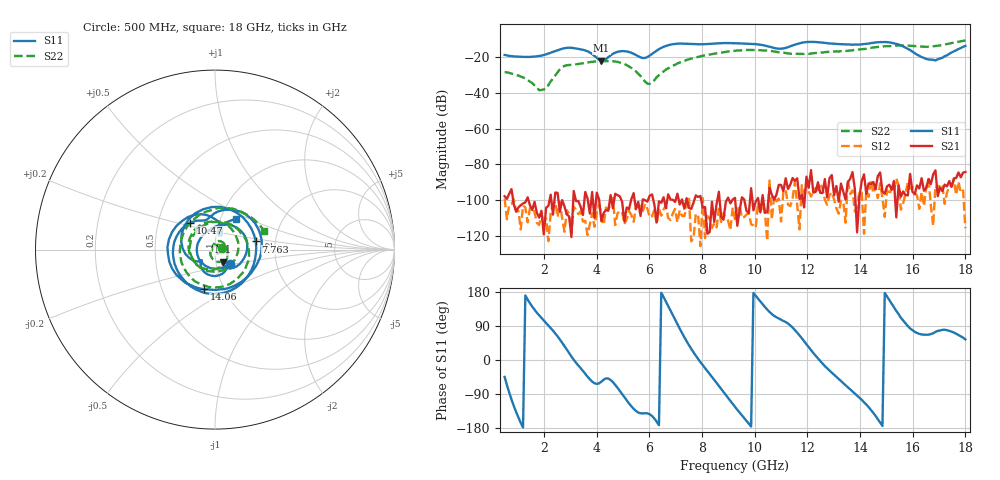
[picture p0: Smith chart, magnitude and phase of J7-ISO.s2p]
!Agilent Technologies,N5230A,MY45001360,A.07.50.67
!Agilent N5230A: A.07.50.67
!Date: Tuesday, April 16, 2024 16:03:02
!Correction: S11(Full 2 Port(1,2))
!S21(Full 2 Port(1,2))
!S12(Full 2 Port(1,2))
!S22(Full 2 Port(1,2))
!S2P File: Measurements: S11, S21, S12, S22:
# Hz S  dB  R 50
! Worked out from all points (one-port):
!   201 points, 500 MHz to 18 GHz, reference 50 ohm
!   lowest |S11| = -22.0 dB at 4.175 GHz (marker M1), VSWR 1.17, Z = 54 - j7.27 ohm
!   |S11| at or under -10 dB: start of sweep to end of sweep
!   S11 on the Smith chart (normalised r, x): 500 MHz: 1.16, -0.19; 7.763 GHz: 1.58, +0.15; 10.47 GHz: 0.73, +0.23; 14.06 GHz: 0.81, -0.38; 18 GHz: 1.19, +0.42
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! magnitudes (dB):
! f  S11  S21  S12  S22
! 500 MHz  -18.7  -97.8  -99.1  -28.4
! 1.288 GHz  -19.9  -101.3  -104.1  -31.9
! 1.9 GHz  -19.1  -106.0  -107.8  -38.4
! 2.075 GHz  -18.4  -104.3  -110.1  -37.7
! 2.688 GHz  -15.3  -100.0  -110.2  -25.6
! 3.475 GHz  -15.9  -108.3  -112.0  -23.4
! 4.175 GHz  -22.0  -111.8  -107.4  -22.3
! 4.7 GHz  -17.5  -96.4  -113.9  -22.4
! 5.05 GHz  -16.7  -111.9  -113.4  -23.8
! 5.487 GHz  -18.8  -105.1  -104.3  -27.9
! 5.925 GHz  -19.9  -100.8  -104.8  -34.8
! 6.362 GHz  -15.5  -100.6  -104.9  -30.1
! 6.888 GHz  -12.8  -99.8  -107.4  -24.8
! 7.763 GHz  -12.7  -97.3  -107.6  -20.1
! 9.25 GHz  -12.2  -98.7  -110.7  -16.5
! 10.47 GHz  -13.8  -106.6  -122.8  -16.4
! 11 GHz  -15.3  -91.5  -111.9  -17.3
! 12.22 GHz  -11.5  -95.8  -94.5  -17.8
! 14.06 GHz  -12.8  -89.3  -95.7  -15.5
! 15.11 GHz  -11.8  -91.4  -97.0  -13.9
! 16.86 GHz  -21.8  -83.3  -92.1  -13.8
! 18 GHz  -13.7  -84.2  -115.7  -10.7
